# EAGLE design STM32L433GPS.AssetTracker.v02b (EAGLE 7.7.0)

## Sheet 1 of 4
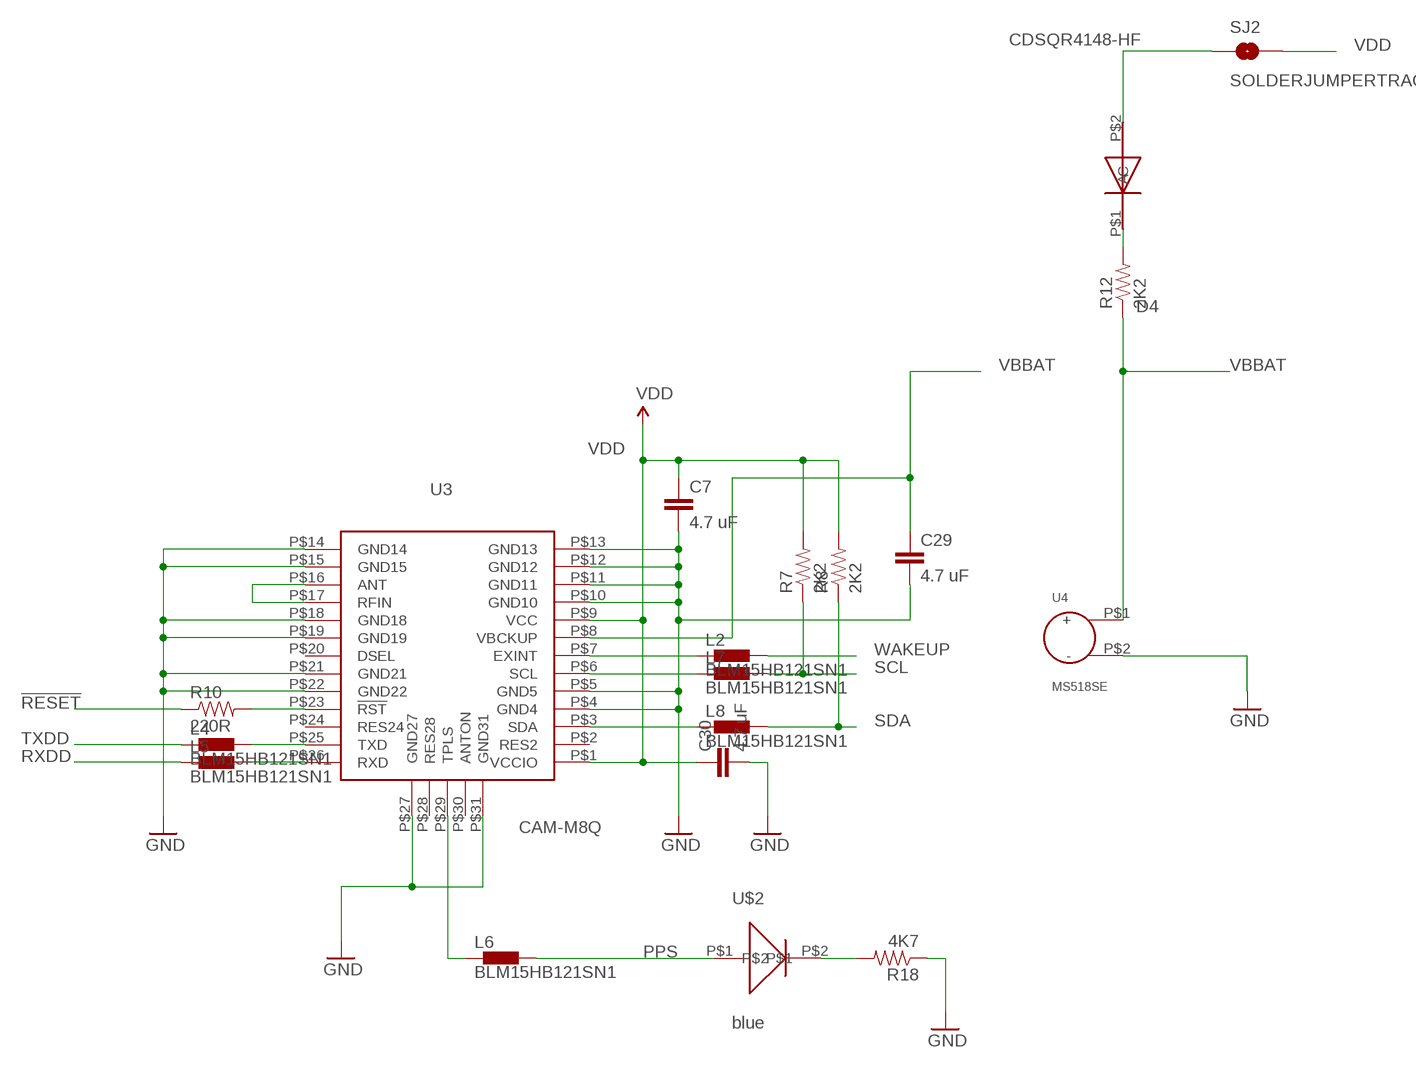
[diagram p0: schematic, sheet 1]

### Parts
C7  4.7 uF  0402CAP.KW  [0402-CAP]
C29  4.7 uF  0402CAP.KW  [0402-CAP]
C30  4.7 uF  0402CAP.KW  [0402-CAP]
D4  CDSQR4148-HF  [CDSQR4148-HF]
L2  BLM15HB121SN1  [0402]
L4  BLM15HB121SN1  [0402]
L5  BLM15HB121SN1  [0402]
L6  BLM15HB121SN1  [0402]
L7  BLM15HB121SN1  [0402]
L8  BLM15HB121SN1  [0402]
R7  2K2  0402RES.KW  [0402-RES]
R8  2K2  0402RES.KW  [0402-RES]
R10  220R  0402RES.KW  [0402-RES]
R12  2K2  0402RES.KW  [0402-RES]
R18  4K7  0402RES.KW  [0402-RES]
SJ2  SOLDERJUMPERTRACE  [SJ_2S-TRACE]
U3  CAM-M8Q  [CAM-M8Q]
U4  MS518SE  [MS518SE]
U$2  blue  0402LED  [0402LED]

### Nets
!RESET: R10.1
GND: C7.2 C29.2 C30.2 R18.1 U3.P$4(GND4) U3.P$5(GND5) U3.P$10(GND10) U3.P$11(GND11) U3.P$12(GND12) U3.P$13(GND13) U3.P$14(GND14) U3.P$15(GND15) U3.P$18(GND18) U3.P$19(GND19) U3.P$21(GND21) U3.P$22(GND22) U3.P$27(GND27) U3.P$31(GND31) U4.P$2(-) ; also sheet 2,3,4
N$4: D4.P$2(A) SJ2.1
N$5: D4.P$1(C) R12.2
N$6: L2.1 U3.P$7(EXINT)
N$8: R18.2 U$2.P$2
N$10: L7.1 U3.P$6(SCL)
N$23: L8.1 U3.P$3(SDA)
N$43: L4.2 U3.P$25(TXD)
N$44: L5.2 U3.P$26(RXD)
N$45: U3.P$16(ANT) U3.P$17(RFIN)
N$46: R10.2 U3.P$23(!RST)
N$47: L6.1 U3.P$29(TPLS)
PPS: L6.2 U$2.P$1 ; also sheet 4
RXDD: L5.1 ; also sheet 4
SCL: L7.2 R7.1 ; also sheet 3,4
SDA: L8.2 R8.1 ; also sheet 3,4
TXDD: L4.1 ; also sheet 4
VBBAT: C29.1 R12.1 U3.P$8(VBCKUP) U4.P$1(+)
VDD: C7.1 C30.1 R7.2 R8.2 SJ2.2 U3.P$1(VCCIO) U3.P$9(VCC) ; also sheet 2,3,4
WAKEUP: L2.2 ; also sheet 4
Unconnected: U3.P$2(RES2) U3.P$20(DSEL) U3.P$24(RES24) U3.P$28(RES28) U3.P$30(ANTON)

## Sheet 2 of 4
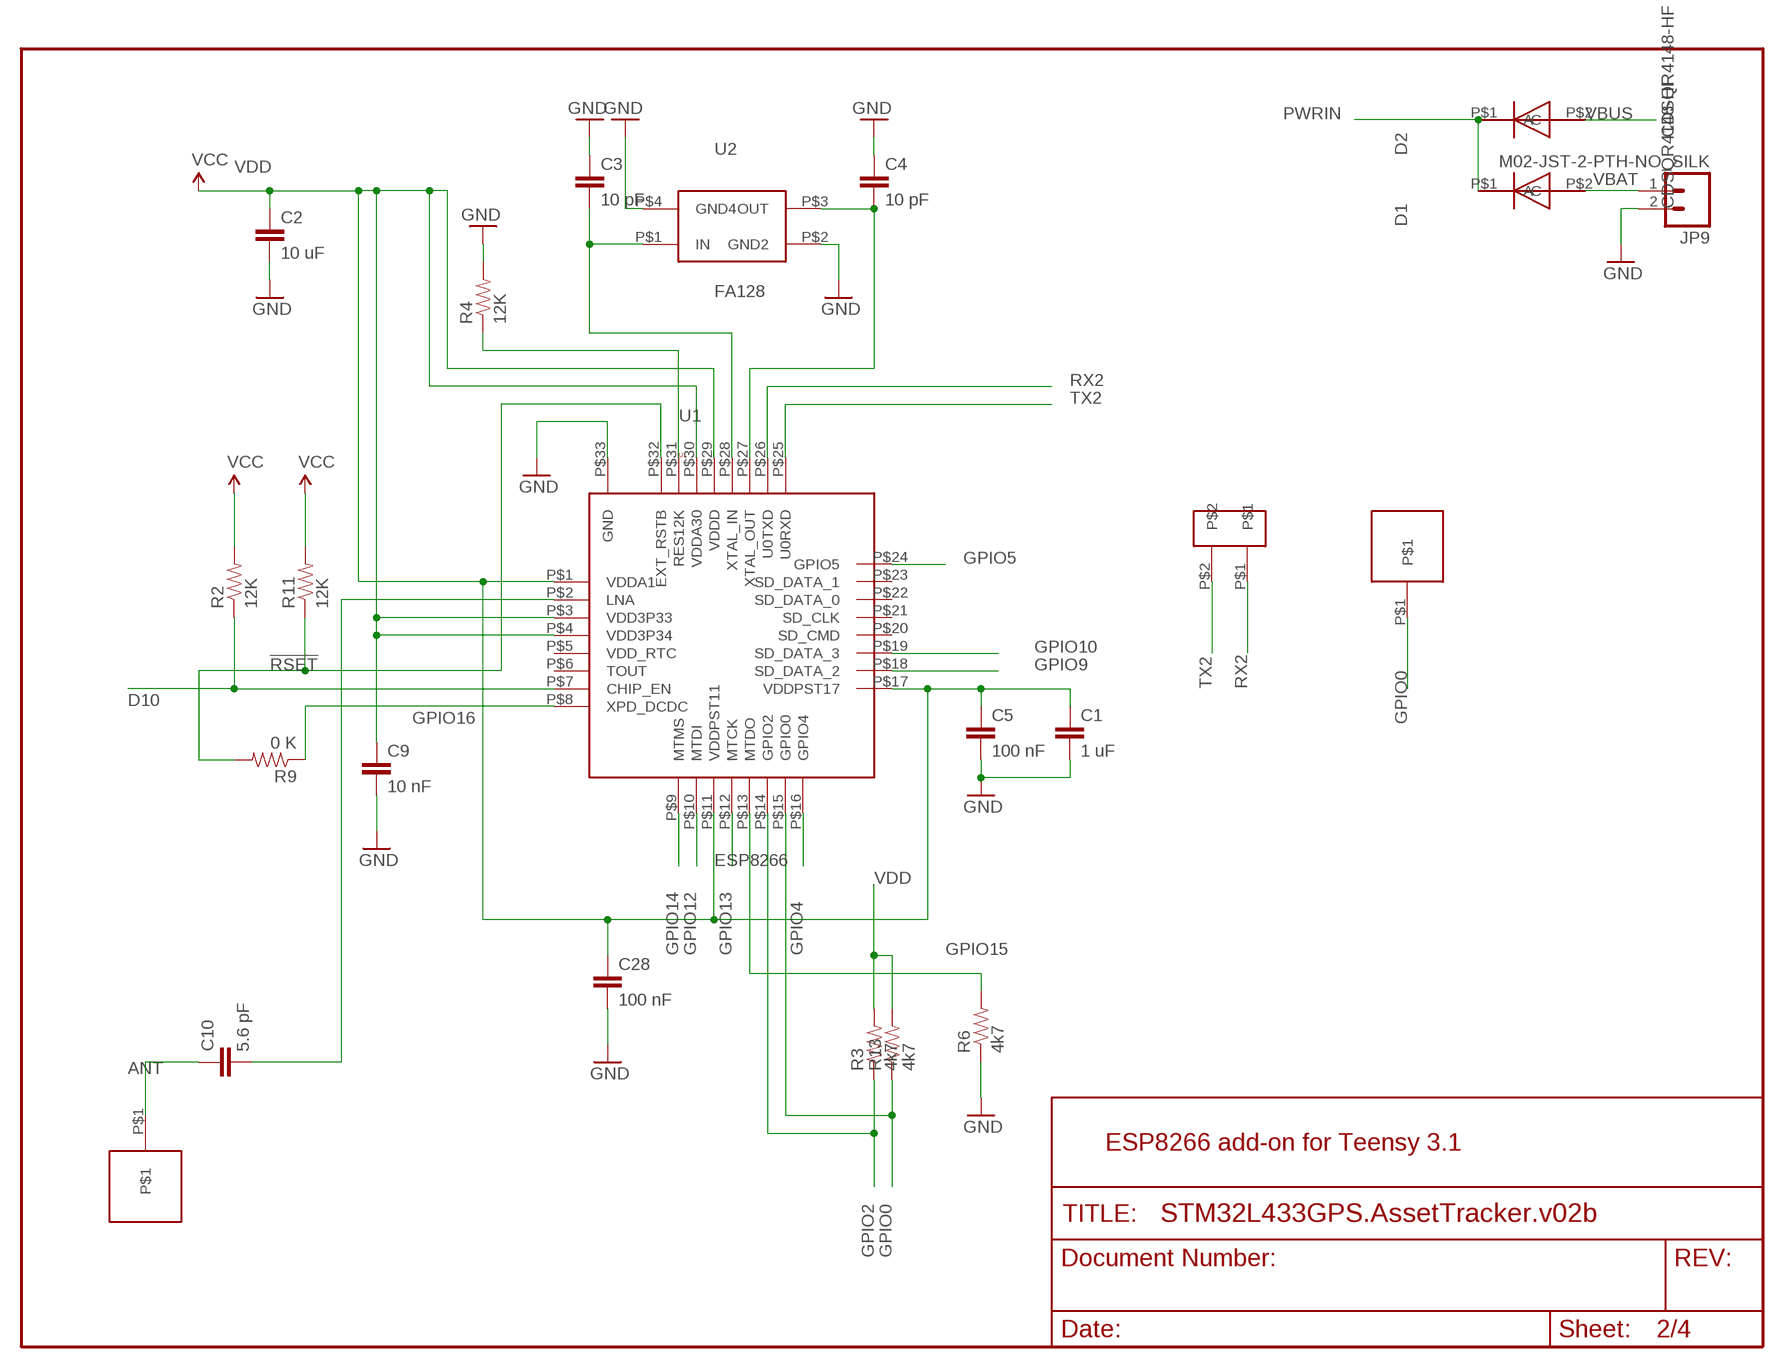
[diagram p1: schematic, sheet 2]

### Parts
C1  1 uF  0402CAP.KW  [0402-CAP]
C2  10 uF  0402CAP.KW  [0402-CAP]
C3  10 pF  0402CAP.KW  [0402-CAP]
C4  10 pF  0402CAP.KW  [0402-CAP]
C5  100 nF  0402CAP.KW  [0402-CAP]
C9  10 nF  0402CAP.KW  [0402-CAP]
C10  5.6 pF  0402CAP.KW  [0402-CAP]
C28  100 nF  0402CAP.KW  [0402-CAP]
D1  CDSQR4148-HF  [CDSQR4148-HF]
D2  CDSQR4148-HF  [CDSQR4148-HF]
JP9  M02-JST-2-PTH-NO_SILK  [JST-2-PTH-NS]
R2  12K  0402RES.KW  [0402-RES]
R3  4k7  0402RES.KW  [0402-RES]
R4  12K  0402RES.KW  [0402-RES]
R6  4k7  0402RES.KW  [0402-RES]
R9  0 K  0402RES.KW  [0402-RES]
R11  12K  0402RES.KW  [0402-RES]
R13  4k7  0402RES.KW  [0402-RES]
U1  ESP8266  [ESP8266]
U2  FA128  [FA128]
U$1  HN02  [HN02]
U$3  HN01  [HN01]
U$15  HN01  [HN01]

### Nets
!RSET: R9.2 R11.1 U1.P$32(EXT_RSTB)
ANT: C10.1 U$15.P$1
D10: R2.1 U1.P$7(CHIP_EN) ; also sheet 4
GND: C1.2 C2.2 C3.1 C4.1 C5.2 C9.2 C28.2 JP9.2 R4.2 R6.1 U1.P$33(GND) U2.P$2(GND2) U2.P$4(GND4) ; also sheet 1,3,4
GPIO0: R13.1 U1.P$15(GPIO0) U$3.P$1
GPIO2: R3.1 U1.P$14(GPIO2)
GPIO4: U1.P$16(GPIO4)
GPIO5: U1.P$24(GPIO5)
GPIO9: U1.P$18(SD_DATA_2)
GPIO10: U1.P$19(SD_DATA_3)
GPIO12: U1.P$10(MTDI)
GPIO13: U1.P$12(MTCK)
GPIO14: U1.P$9(MTMS)
GPIO15: R6.2 U1.P$13(MTDO)
GPIO16: R9.1 U1.P$8(XPD_DCDC)
N$1: C3.2 U1.P$28(XTAL_IN) U2.P$1(IN)
N$2: C4.2 U1.P$27(XTAL_OUT) U2.P$3(OUT)
N$3: C10.2 U1.P$2(LNA)
N$13: R4.1 U1.P$31(RES12K)
PWRIN: D1.P$1(C) D2.P$1(C) ; also sheet 4
RX2: U1.P$26(U0TXD) U$1.P$1 ; also sheet 4
TX2: U1.P$25(U0RXD) U$1.P$2 ; also sheet 4
VBAT: D1.P$2(A) JP9.1 ; also sheet 4
VBUS: D2.P$2(A) ; also sheet 4
VDD: C1.1 C2.1 C5.1 C9.1 C28.1 R2.2 R3.2 R11.2 R13.2 U1.P$1(VDDA1) U1.P$3(VDD3P33) U1.P$4(VDD3P34) U1.P$11(VDDPST11) U1.P$17(VDDPST17) U1.P$29(VDDD) U1.P$30(VDDA30) ; supply symbol labelled VCC ; also sheet 1,3,4
Unconnected: U1.P$5(VDD_RTC) U1.P$6(TOUT) U1.P$20(SD_CMD) U1.P$21(SD_CLK) U1.P$22(SD_DATA_0) U1.P$23(SD_DATA_1)

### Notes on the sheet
- ESP8266 add-on for Teensy 3.1

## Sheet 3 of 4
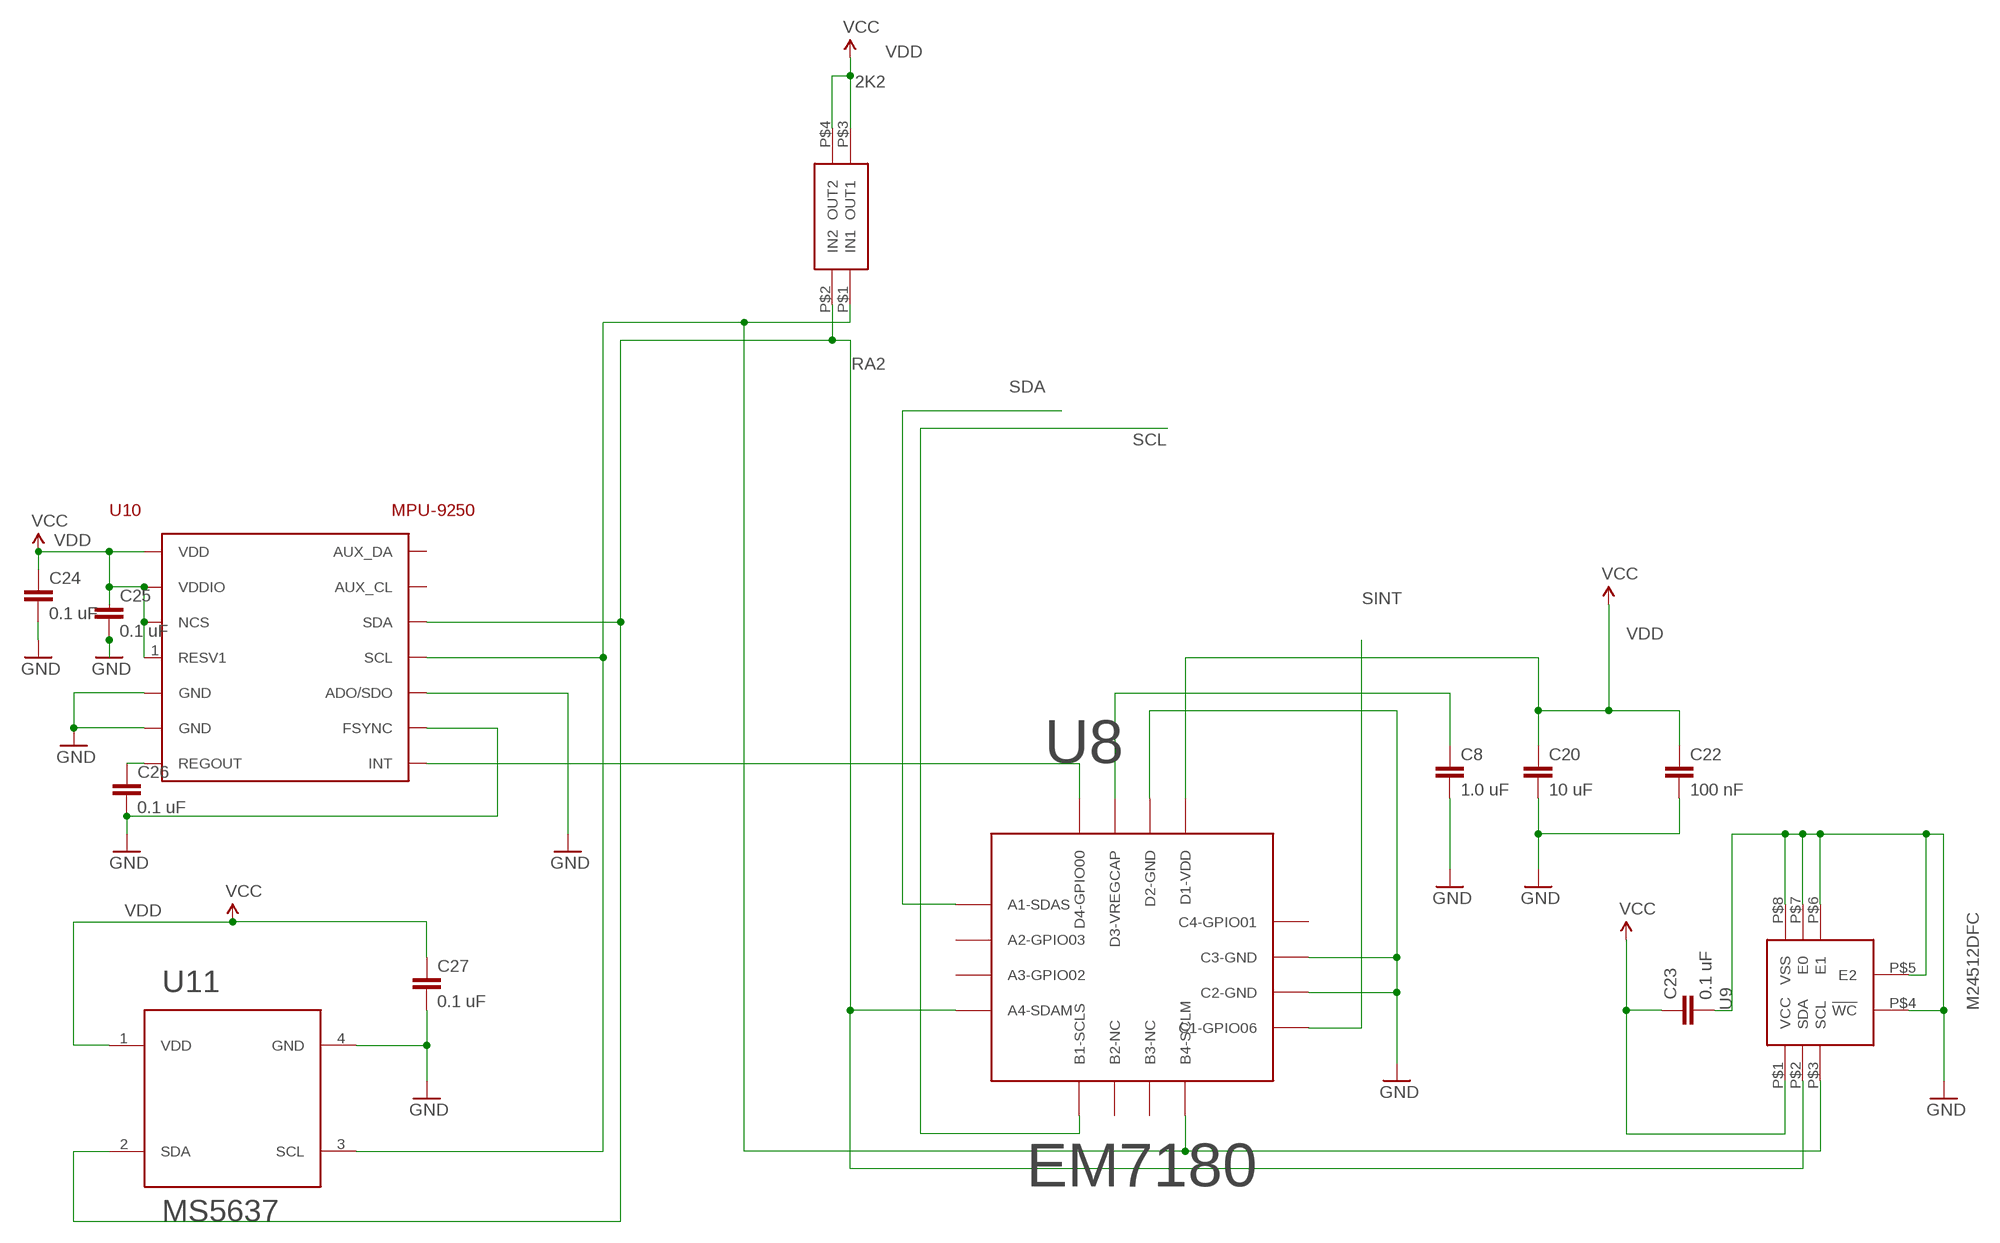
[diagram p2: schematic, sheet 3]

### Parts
C8  1.0 uF  CAP0402-CAP  [0402-CAP]
C20  10 uF  CAP0402-CAP  [0402-CAP]
C22  100 nF  CAP0402-CAP  [0402-CAP]
C23  0.1 uF  CAP0402-CAP  [0402-CAP]
C24  0.1 uF  CAP0402-CAP  [0402-CAP]
C25  0.1 uF  CAP0402-CAP  [0402-CAP]
C26  0.1 uF  CAP0402-CAP  [0402-CAP]
C27  0.1 uF  CAP0402-CAP  [0402-CAP]
RA2  2K2  EXB24V  [EXB24V]
U8  EM7180  [WL-CSP16]
U9  M24512DFC  [M24512DFC]
U10  MPU-9250  [MPU-9250]
U11  MS5637  [MS5637QFN-4]

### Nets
GND: C8.2 C20.2 C22.2 C23.2 C24.2 C25.2 C26.2 C27.2 U8.P$10(C2-GND) U8.P$11(C3-GND) U8.P$14(D2-GND) U9.P$4(!WC) U9.P$5(E2) U9.P$6(E1) U9.P$7(E0) U9.P$8(VSS) U10.9(ADO/SDO) U10.11(FSYNC) U10.18(GND) U10.20(GND) U11.4(GND) ; also sheet 1,2,4
N$19: U8.P$16(D4-GPIO00) U10.12(INT)
N$26: C8.1 U8.P$15(D3-VREGCAP)
N$40: C26.1 U10.10(REGOUT)
SCL: U8.P$5(B1-SCLS) ; also sheet 1,4
SCL2: RA2.P$1(IN1) U8.P$8(B4-SCLM) U9.P$3(SCL) U10.23(SCL) U11.3(SCL)
SDA: U8.P$1(A1-SDAS) ; also sheet 1,4
SDA2: RA2.P$2(IN2) U8.P$4(A4-SDAM) U9.P$2(SDA) U10.24(SDA) U11.2(SDA)
SINT: U8.P$9(C1-GPIO06) ; also sheet 4
VDD: C20.1 C22.1 C23.1 C24.1 C25.1 C27.1 RA2.P$3(OUT1) RA2.P$4(OUT2) U8.P$13(D1-VDD) U9.P$1(VCC) U10.1(RESV1) U10.8(VDDIO) U10.13(VDD) U10.22(NCS) U11.1(VDD) ; supply symbol labelled VCC ; also sheet 1,2,4
Unconnected: U8.P$2(A2-GPIO03) U8.P$3(A3-GPIO02) U8.P$6(B2-NC) U8.P$7(B3-NC) U8.P$12(C4-GPIO01) U10.7(AUX_CL) U10.21(AUX_DA)

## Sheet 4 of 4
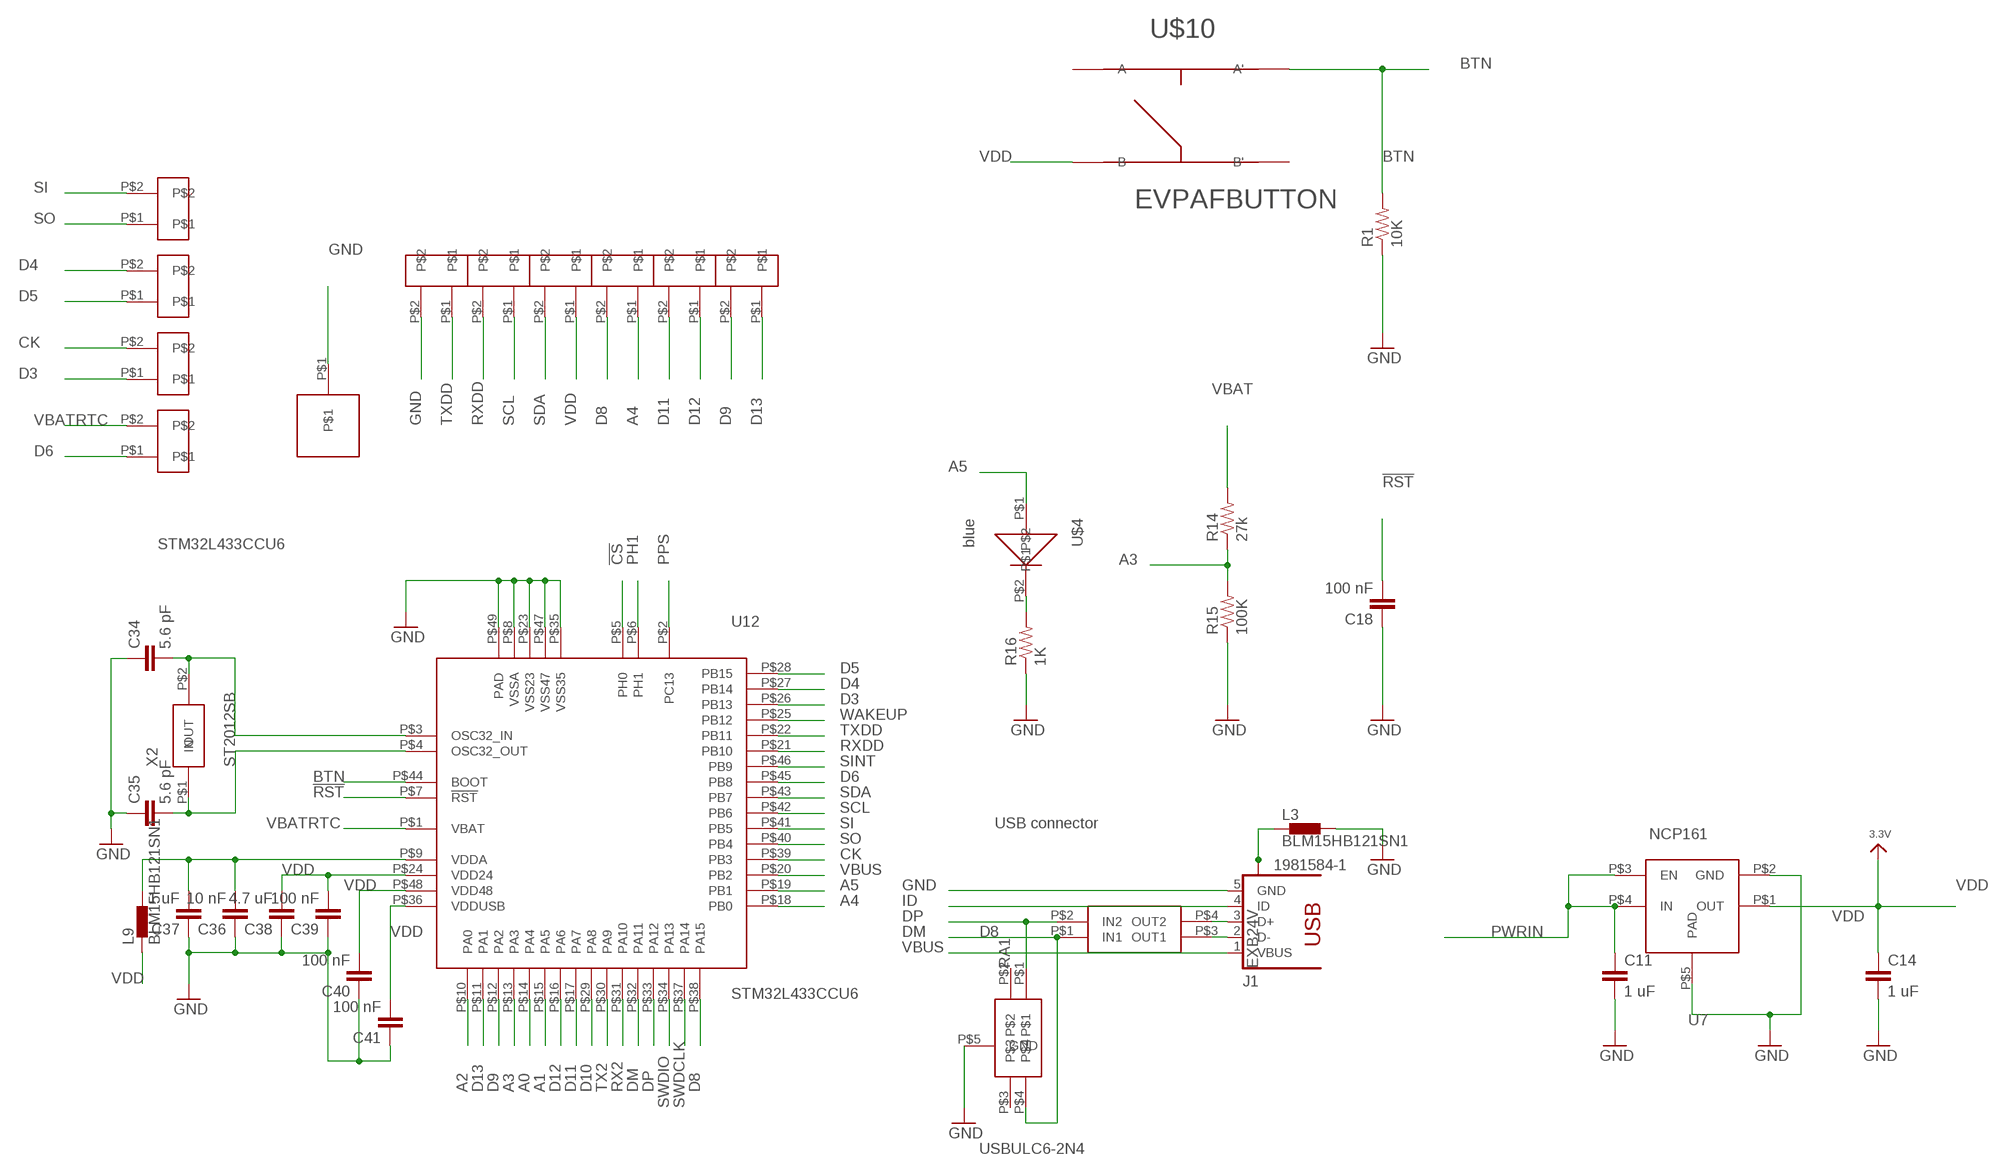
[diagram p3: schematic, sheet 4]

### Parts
C11  1 uF  CAP0402-CAP  [0402-CAP]
C14  1 uF  CAP0402-CAP  [0402-CAP]
C18  100 nF  0402CAP.KW  [0402-CAP]
C34  5.6 pF  0402CAP.KW  [0402-CAP]
C35  5.6 pF  0402CAP.KW  [0402-CAP]
C36  10 nF  0402CAP.KW  [0402-CAP]
C37  1 uF  0402CAP.KW  [0402-CAP]
C38  4.7 uF  0402CAP.KW  [0402-CAP]
C39  100 nF  0402CAP.KW  [0402-CAP]
C40  100 nF  0402CAP.KW  [0402-CAP]
C41  100 nF  0402CAP.KW  [0402-CAP]
D8  USBULC6-2N4  [USBULC6-2N4]
J1  1981584-1  [1981584-1]
L3  BLM15HB121SN1  [0402]
L9  BLM15HB121SN1  [0402]
R1  10K  0402RES.KW  [0402-RES]
R14  27k  0402RES.KW  [0402-RES]
R15  100K  0402RES.KW  [0402-RES]
R16  1K  0402RES.KW  [0402-RES]
RA1  EXB24V  [EXB24V]
U7  NCP161  [NCP161]
U12  STM32L433CCU6  [STM32L433CCU6]
U$4  blue  0402LED  [0402LED]
U$10  EVPAFBUTTON  [EVPAF-BUTTON-SPDT]
U$11  HN02  [HN02]
U$12  HN02  [HN02]
U$13  HN02  [HN02]
U$14  HN02  [HN02]
U$16  HN02  [HN02]
U$17  HN02  [HN02]
U$19  HN01  [HN01]
U$30  HN02  [HN02]
U$31  HN02  [HN02]
U$32  HN02  [HN02]
U$36  HN02  [HN02]
X2  ST2012SB  [ST2012SB]

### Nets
!CS: U12.P$5(PH0)
!RST: C18.2 U12.P$7(!RST)
A0: U12.P$14(PA4)
A1: U12.P$15(PA5)
A2: U12.P$10(PA0)
A3: R14.1 R15.2 U12.P$13(PA3)
A4: U12.P$18(PB0) U$14.P$1
A5: U12.P$19(PB1) U$4.P$1
BTN: R1.2 U12.P$44(BOOT) U$10.P$2(A')
CK: U12.P$39(PB3) U$31.P$2
D3: U12.P$26(PB13) U$31.P$1
D4: U12.P$27(PB14) U$32.P$2
D5: U12.P$28(PB15) U$32.P$1
D6: U12.P$45(PB8) U$36.P$1
D8: U12.P$38(PA15) U$14.P$2
D9: U12.P$12(PA2) U$16.P$2
D10: U12.P$29(PA8) ; also sheet 2
D11: U12.P$17(PA7) U$17.P$2
D12: U12.P$16(PA6) U$17.P$1
D13: U12.P$11(PA1) U$16.P$1
DM: D8.P$4 RA1.P$1(IN1) U12.P$32(PA11)
DP: D8.P$1 RA1.P$2(IN2) U12.P$33(PA12)
GND: C11.2 C14.2 C18.1 C34.1 C35.1 C36.1 C37.1 C38.1 C39.1 C40.1 C41.1 D8.P$5(GND) J1.5(GND) L3.2 R1.1 R15.1 R16.1 U7.P$2(GND) U7.P$5(PAD) U12.P$8(VSSA) U12.P$23(VSS23) U12.P$35(VSS35) U12.P$47(VSS47) U12.P$49(PAD) U$11.P$2 U$19.P$1 ; also sheet 1,2,3
ID: J1.4(ID)
N$9: C34.2 U12.P$3(OSC32_IN) X2.P$2(OUT)
N$11: R16.2 U$4.P$2
N$12: C35.2 U12.P$4(OSC32_OUT) X2.P$1(IN)
N$17: C36.2 C37.2 L9.2 U12.P$9(VDDA)
N$31: J1.3(D+) RA1.P$4(OUT2)
N$33: J1.2(D-) RA1.P$3(OUT1)
PH1: U12.P$6(PH1)
PPS: U12.P$2(PC13) ; also sheet 1
PWRIN: C11.1 U7.P$3(EN) U7.P$4(IN) ; also sheet 2
RX2: U12.P$31(PA10) ; also sheet 2
RXDD: U12.P$21(PB10) U$12.P$2 ; also sheet 1
SCL: U12.P$42(PB6) U$12.P$1 ; also sheet 1,3
SDA: U12.P$43(PB7) U$13.P$2 ; also sheet 1,3
SI: U12.P$41(PB5) U$30.P$2
SINT: U12.P$46(PB9) ; also sheet 3
SO: U12.P$40(PB4) U$30.P$1
SWDCLK: U12.P$37(PA14)
SWDIO: U12.P$34(PA13)
TX2: U12.P$30(PA9) ; also sheet 2
TXDD: U12.P$22(PB11) U$11.P$1 ; also sheet 1
USB_SHIELD1: J1.S1 J1.S2 J1.S3 J1.S4 L3.1
VBAT: R14.2 ; also sheet 2
VBATRTC: U12.P$1(VBAT) U$36.P$2
VBUS: J1.1(VBUS) U12.P$20(PB2) ; also sheet 2
VDD: C14.1 C38.2 C39.2 C40.2 C41.2 L9.1 U7.P$1(OUT) U12.P$24(VDD24) U12.P$36(VDDUSB) U12.P$48(VDD48) U$10.P$3(B) U$13.P$1 ; supply symbol labelled 3.3V ; also sheet 1,2,3
WAKEUP: U12.P$25(PB12) ; also sheet 1
Unconnected: D8.P$2 D8.P$3 U$10.P$1(A) U$10.P$4(B')

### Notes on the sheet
- STM32L433CCU6
- USB connector

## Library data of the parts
C1-C5 C7 C9 C10 C18 C28-C30 C34-C41 = SparkFun-Capacitors:0402CAP.KW
C8 C11 C14 C20 C22-C27 = SparkFun-Capacitors:CAP: Capacitor
D1 D2 D4 = Kris:CDSQR4148-HF: ComChip's CDSQR4148-HF high speed 150 mA Io diode
D8 = Kris:USBULC6-2N4: ST TVS diode ESD Protection USBULC6-2N4
J1 = con-usb:1981584-1: Receptacle, micro-USB, type A/B Tyco Electronics; MF: Hirose; MPN: ZX62-AB-5PA(11)
JP9 = SparkFun-Connectors:M02: Standard 2-pin 0.1" header. Use with
L2-L9 = inductors:BLM15H: EMIFIL (R) Chip Ferrite Bead for GHz Noise
R1-R4 R6-R16 R18 = SparkFun-Resistors:0402RES.KW
RA1 RA2 = Kris:EXB24V: Panasonic EXB24 22 Ohm series resistor pair
SJ2 = SparkFun-Passives:SOLDERJUMPER: Solder Jumper
U1 = Kris:ESP8266: QFN-32 package for espressif's ESP8266 WiFi microprocessor
U2 = Kris:FA128: FA-128 Espon crystal
U3 = ubloxLib:CAM-M8Q: CAM-M8Q GPS/GNSS Module https://www.u-blox.com/sites/default/files/CAM-M8_HardwareIntegrationManual_%28UBX-14000014%29.pdf
U4 = Kris:MS518SE: S518SE 3 V rechargable Li battery
U7 = Kris:NCP161: NCP161 3V3 LDO voltage regulator
U8 = SparkFun-DigitalIC:EM7180: WL-CSP19 package for the EM7180 SENtral sensor fusion hub
U9 = Kris:M24512DFC: ST's M24512DFC6 512 Mbit EEPROM
U10 = SparkFun-Sensors:MPU-9250: The MPU-9250 is a 9-axis motion sensor that contains an accelerometer/gyro sensor (MPU-6500) combined with a magnetometer (AK8963).
U11 = SparkFun-DiscreteSemi:MS5637: MS5637 I2C pressure sensor in QFN-4 package by Measurement Specialties
U12 = STM32L433CCU6:STM32L433CCU6: UFQFPN48 48-lead, 7 mm x 7 mm, 0.5-mm pitch, ultra thin fine pitch quad flat package for STM32L433 http://www.st.com/content/ccc/resource/technical/document/datasheet/f7/a0/fc/27/24/4e/4f/3f/DM00257192.pdf/files/DM00257192.pdf/jcr:content/translations/en.DM00257192.pdf
U$1 U$11-U$14 U$16 U$17 U$30-U$32 U$36 = Kris:HN02: 0.1 inch header
U$2 U$4 = Kris:0402LED: 0402led
U$3 U$15 U$19 = PWSONN6:HN01
U$10 = SparkFun-Electromechanical:EVPAFBUTTON: EVPAF Momentary switch by panasonic
X2 = Kris:ST2012SB: Kyocera 2.0 x 1.2 mm 32.768 20kHz ppm 4 pf crystal

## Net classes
1 USB: width 0.254 mm, drill 0.33 mm, clearance 0.159 mm
2 Top GND Pour: clearance 0.762 mm to class 1

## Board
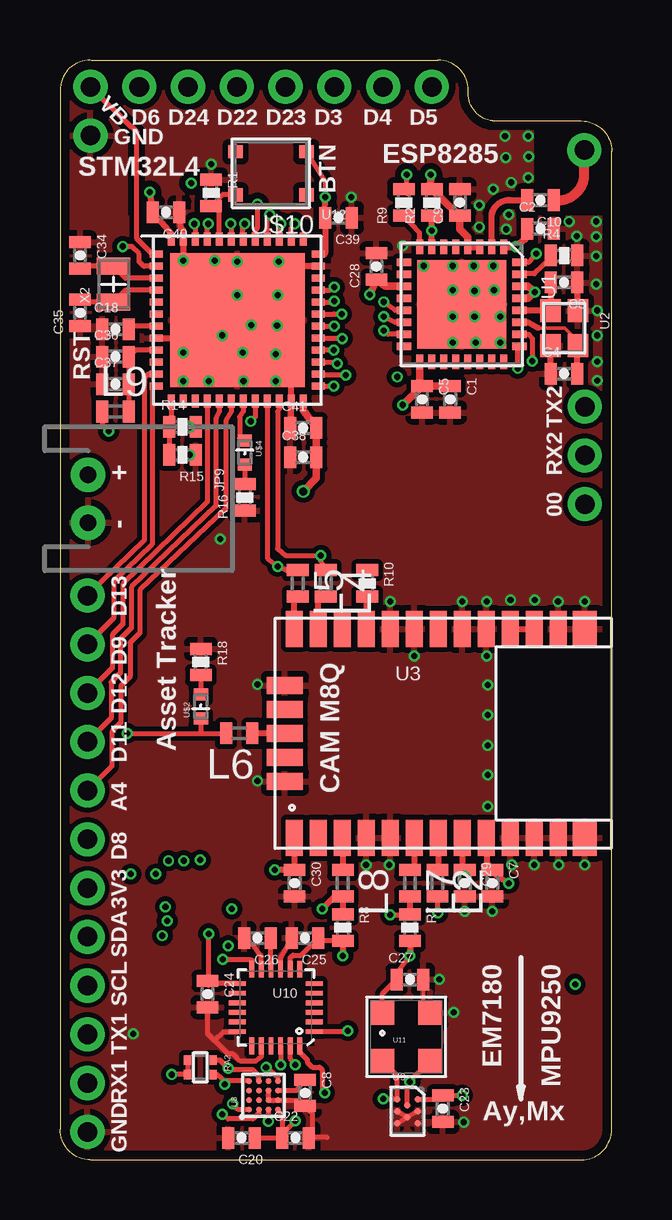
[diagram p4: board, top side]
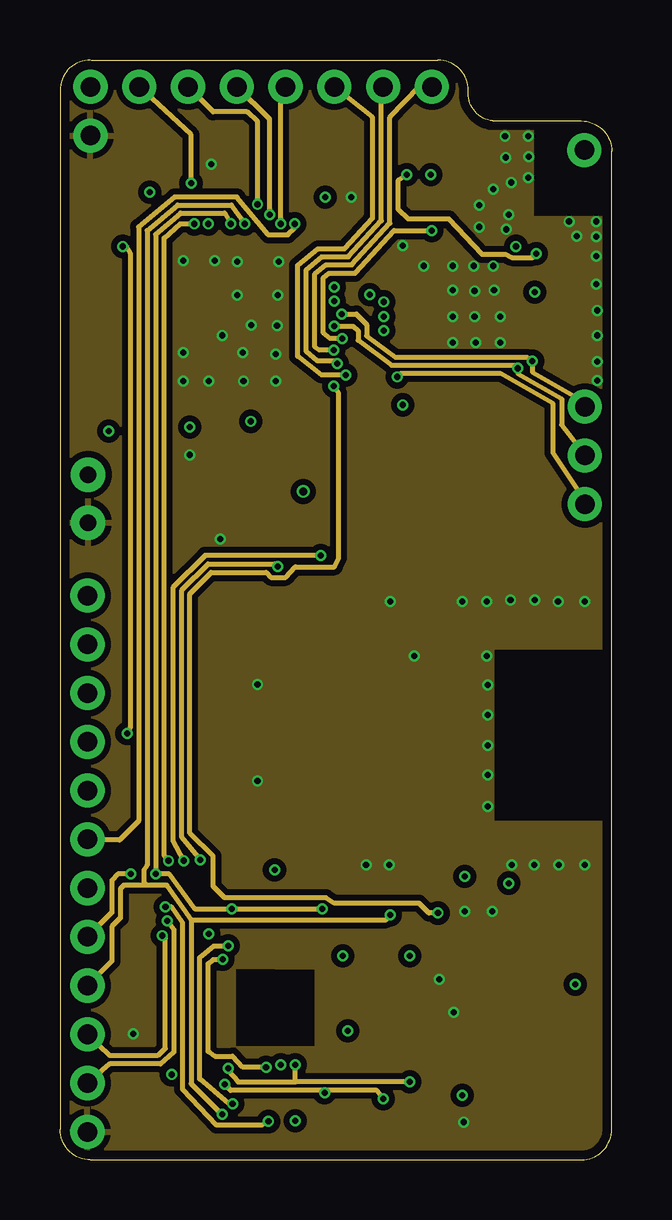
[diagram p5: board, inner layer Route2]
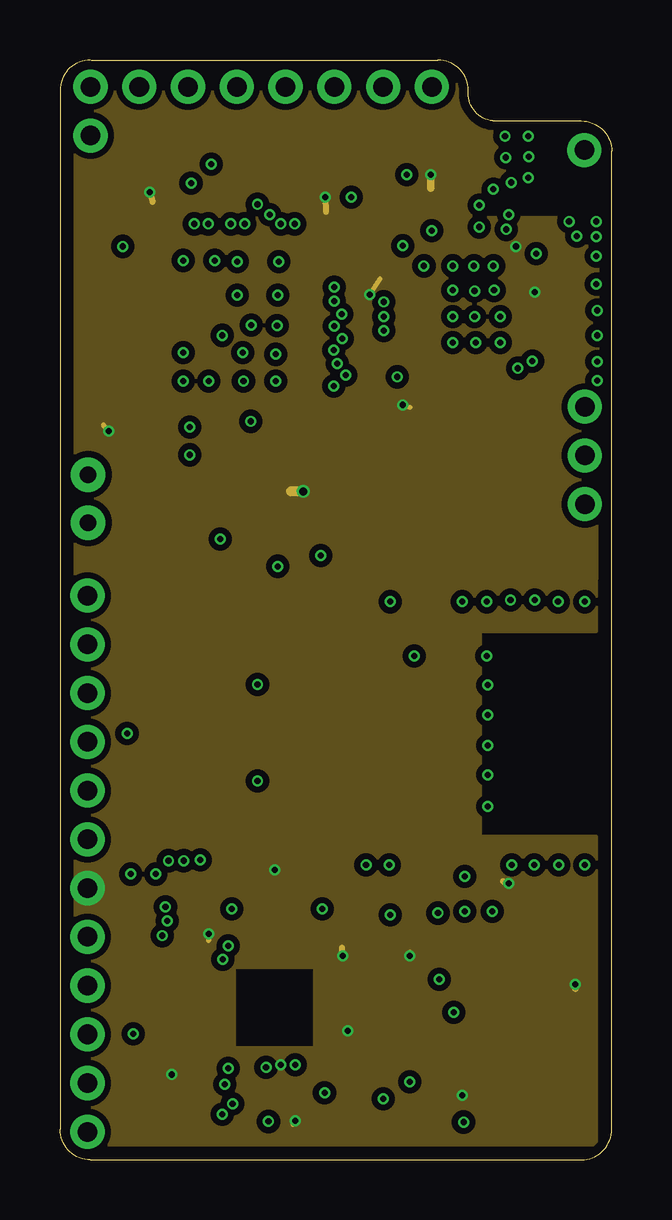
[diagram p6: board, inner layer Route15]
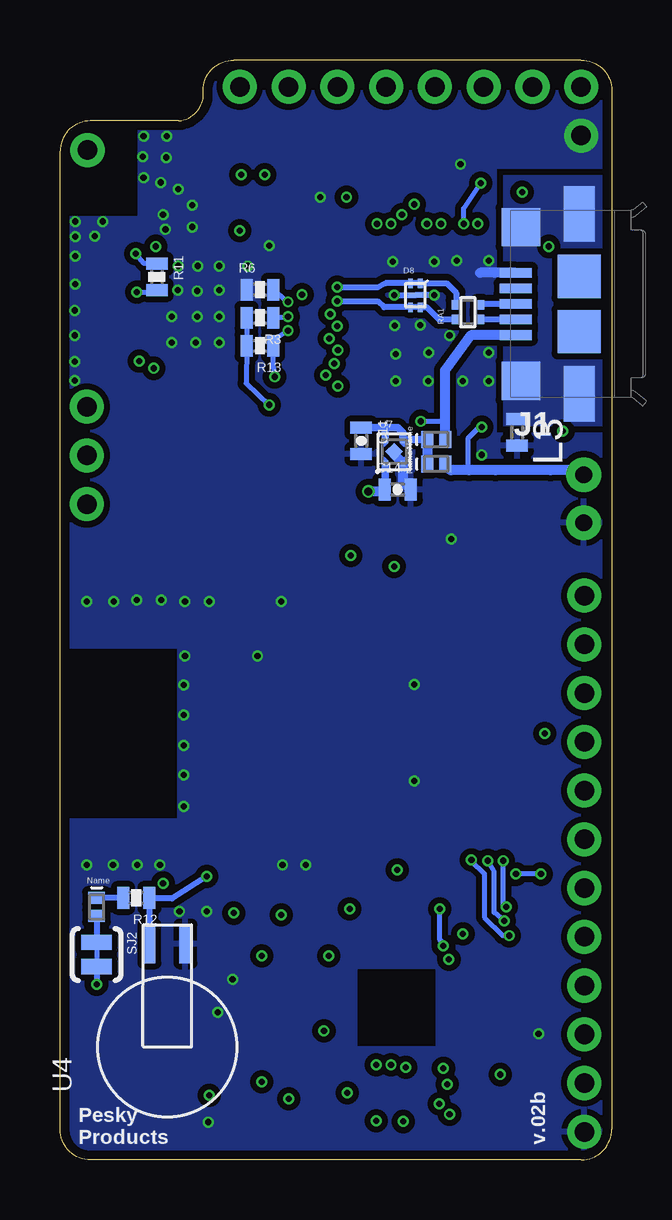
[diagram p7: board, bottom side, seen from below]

Size 22.99 x 45.85 mm. Coordinates in mm from the lower left corner, seen from the top.
Outline: 1.27,45.85 arc90 0,44.58 0,1.27 arc90 1.27,0 21.72,0 arc90 22.99,1.27 22.99,42.04 arc90 21.72,43.31 18.03,43.31 arc-90 17.02,44.58 arc90 15.75,45.85 1.29,45.85
Copper layers (1*2*15*16): Top 0.035559375mm / dielectric 0.17018125mm / Route2 0.01778125mm / dielectric 47mil / Route15 0.01778125mm / dielectric 0.17018125mm / Bottom 0.035559375mm
Design rules "OSHPark-4layer *": minimum track width 5mil, minimum drill 10mil, track to track 5mil, track to pad 5mil, pad to pad 5mil, via to via 5mil, smd to smd 5mil, copper to edge 15mil, drill to drill 6mil, minimum pad ring 4mil, minimum via ring 4mil, stop-mask expansion 4mil, vias tented up to drill 20mil, thermal gap 10mil

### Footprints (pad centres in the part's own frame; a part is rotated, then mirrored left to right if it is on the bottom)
0402-CAP = smd 0.5 x 0.9: 1 -0.55,0; 2 0.55,0
CDSQR4148-HF = smd 0.7 x 0.5: P$1 0,0.375; P$2 0,-0.375
USBULC6-2N4 = smd 0.2 x 0.4: P$1 0.2,0.5; P$2 -0.2,0.5; P$3 -0.2,-0.5; P$4 0.2,-0.5 | smd 0.6 x 0.2: P$5 0,0
1981584-1 = smd 0.4 x 1.35: 1 -1.3,4.1; 2 -0.65,4.1; 3 0,4.1; 4 0.65,4.1; 5 1.3,4.1 | smd 1.8 x 1.8: M1 -1.15,1.45; M2 1.15,1.45 | smd 2.3 x 1.3: S1 -3.75,1.45; S2 3.75,1.45 | smd 1.6 x 1.6: S3 -3.2,3.885; S4 3.2,3.885
JST-2-PTH-NS = drill 0.7 pad 1.448: 1 -1,0; 2 1,0
0402 = smd 0.5 x 0.9: 1 -0.55,0; 2 0.55,0
0402-RES = smd 0.5 x 0.9: 1 -0.55,0; 2 0.55,0
EXB24V = smd 0.4 x 0.36: P$1 -0.3,0.5; P$2 0.3,0.5; P$3 -0.3,-0.5; P$4 0.3,-0.5
SJ_2S-TRACE = smd 0.635 x 1.27: 1 -0.508,0; 2 0.508,0
ESP8266 = smd 0.6 x 0.3: P$1 -2.4,1.75; P$2 -2.4,1.25; P$3 -2.4,0.75; P$4 -2.4,0.25; P$5 -2.4,-0.25; P$6 -2.4,-0.75; P$7 -2.4,-1.25; P$8 -2.4,-1.75; P$17 2.4,-1.75; P$18 2.4,-1.25; P$19 2.4,-0.75; P$20 2.4,-0.25; P$21 2.4,0.25; P$22 2.4,0.75; P$23 2.4,1.25; P$24 2.4,1.75 | smd 0.3 x 0.6: P$9 -1.75,-2.4; P$10 -1.25,-2.4; P$11 -0.75,-2.4; P$12 -0.25,-2.4; P$13 0.25,-2.4; P$14 0.75,-2.4; P$15 1.25,-2.4; P$16 1.75,-2.4; P$25 1.75,2.4; P$26 1.25,2.4; P$27 0.75,2.4; P$28 0.25,2.4; P$29 -0.25,2.4; P$30 -0.75,2.4; P$31 -1.25,2.4; P$32 -1.75,2.4 | smd 3.7 x 3.7: P$33 0,0
FA128 = smd 0.95 x 0.85: P$1 -0.725,-0.575; P$2 0.725,-0.575; P$3 0.725,0.575; P$4 -0.725,0.575
CAM-M8Q = smd 0.7 x 1.5: P$1 0.8,0.45; P$2 1.8,0.45; P$3 2.8,0.45; P$4 3.8,0.45; P$5 4.8,0.45; P$6 5.8,0.45; P$7 6.8,0.45; P$8 7.8,0.45; P$9 8.8,0.45; P$10 9.8,0.45; P$11 10.8,0.45; P$12 11.8,0.45; P$15 11.8,9.15; P$16 10.8,9.15; P$17 9.8,9.15; P$18 8.8,9.15; P$19 7.8,9.15; P$20 6.8,9.15; P$21 5.8,9.15; P$22 4.8,9.15; P$23 3.8,9.15; P$24 2.8,9.15; P$25 1.8,9.15; P$26 0.8,9.15 | smd 1 x 1.5: P$13 12.9,0.45; P$14 12.9,9.15 | smd 1.5 x 0.7: P$27 0.4,6.8; P$28 0.4,5.8; P$29 0.4,4.8; P$30 0.4,3.8; P$31 0.4,2.8
MS518SE = smd 1.6 x 0.5: P$1 4.3,0.75; P$2 4.3,-0.75
NCP161 = smd 0.24 x 0.24: P$1 -0.37,-0.48; P$2 0.37,-0.48; P$3 0.37,0.48; P$4 -0.37,0.48 | smd 0.52 x 0.52 rotated 45: P$5 0,0
WL-CSP16 = smd 0.24 x 0.24: P$1 -0.6,0.6; P$2 -0.2,0.6; P$3 0.2,0.6; P$4 0.6,0.6; P$5 -0.6,0.2; P$6 -0.2,0.2; P$7 0.2,0.2; P$8 0.6,0.2; P$9 -0.6,-0.2; P$10 -0.2,-0.2; P$11 0.2,-0.2; P$12 0.6,-0.2; P$13 -0.6,-0.6; P$14 -0.2,-0.6; P$15 0.2,-0.6; P$16 0.6,-0.6
M24512DFC = smd 0.27 x 0.27: P$1 0.433,0.5; P$2 -0.433,0.5; P$3 0,0.25; P$4 0.433,0; P$5 -0.433,0; P$6 0,-0.25; P$7 0.433,-0.5; P$8 -0.433,-0.5
MPU-9250 = smd 0.7 x 0.2: 1 -1.6,1; 2 -1.6,0.6; 3 -1.6,0.2; 4 -1.6,-0.2; 5 -1.6,-0.6; 6 -1.6,-1; 13 1.6,-1; 14 1.6,-0.6; 15 1.6,-0.2; 16 1.6,0.2; 17 1.6,0.6; 18 1.6,1 | smd 0.2 x 0.7: 7 -1,-1.6; 8 -0.6,-1.6; 9 -0.2,-1.6; 10 0.2,-1.6; 11 0.6,-1.6; 12 1,-1.6; 19 1,1.6; 20 0.6,1.6; 21 0.2,1.6; 22 -0.2,1.6; 23 -0.6,1.6; 24 -1,1.6
MS5637QFN-4 = smd 1 x 1: 1 -1,1; 2 -1,-1; 3 1,-1; 4 1,1
STM32L433CCU6 = smd 0.55 x 0.3: P$1 -3.375,2.75; P$2 -3.375,2.25; P$3 -3.375,1.75; P$4 -3.375,1.25; P$5 -3.375,0.75; P$6 -3.375,0.25; P$7 -3.375,-0.25; P$8 -3.375,-0.75; P$9 -3.375,-1.25; P$10 -3.375,-1.75; P$11 -3.375,-2.25; P$12 -3.375,-2.75; P$25 3.375,-2.75; P$26 3.375,-2.25; P$27 3.375,-1.75; P$28 3.375,-1.25; P$29 3.375,-0.75; P$30 3.375,-0.25; P$31 3.375,0.25; P$32 3.375,0.75; P$33 3.375,1.25; P$34 3.375,1.75; P$35 3.375,2.25; P$36 3.375,2.75 | smd 0.3 x 0.55: P$13 -2.75,-3.375; P$14 -2.25,-3.375; P$15 -1.75,-3.375; P$16 -1.25,-3.375; P$17 -0.75,-3.375; P$18 -0.25,-3.375; P$19 0.25,-3.375; P$20 0.75,-3.375; P$21 1.25,-3.375; P$22 1.75,-3.375; P$23 2.25,-3.375; P$24 2.75,-3.375; P$37 2.75,3.375; P$38 2.25,3.375; P$39 1.75,3.375; P$40 1.25,3.375; P$41 0.75,3.375; P$42 0.25,3.375; P$43 -0.25,3.375; P$44 -0.75,3.375; P$45 -1.25,3.375; P$46 -1.75,3.375; P$47 -2.25,3.375; P$48 -2.75,3.375 | smd 5.6 x 5.6: P$49 0,0
HN02 = drill 0.813 pad 1.422: P$1 0,0; P$2 -2.032,0
0402LED = smd 0.5 x 0.6: P$1 -0.5,0; P$2 0.5,0
HN01 = drill 0.813 pad 1.422: P$1 0,0
EVPAF-BUTTON-SPDT = smd 0.6 x 0.55: P$1 -1.475,0.9; P$2 1.475,0.9; P$3 -1.475,-0.9; P$4 1.475,-0.9
ST2012SB = smd 0.7 x 1.4: P$1 -0.75,0; P$2 0.75,0

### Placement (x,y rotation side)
C1  16.26,31.7 270 top
C2  20.02,38.81 0 top
C3  21.01,36.58 180 top
C4  21.01,32.77 0 top
C5  15.09,31.7 270 top
C7  18.01,11.53 270 top
C8  10.21,2.79 270 top
C9  16.66,39.9 90 top
C10  20.02,40.01 180 top
C11  10.44,29.97 270 bottom
C14  8.92,27.94 0 bottom
C18  2.31,34.62 0 top
C20  7.57,0.91 180 top
C22  9.8,0.91 0 top
C23  15.95,2.13 270 top
C24  6.15,6.91 270 top
C25  10.21,9.25 180 top
C26  8.23,9.25 180 top
C27  14.58,7.52 0 top
C28  13.18,37.24 90 top
C29  16.87,11.53 270 top
C30  9.78,11.53 270 top
C34  0.84,37.69 270 top
C35  0.84,35.31 90 top
C36  2.31,33.48 0 top
C37  2.31,32.33 0 top
C38  10.13,29.29 0 top
C39  11.61,39.27 180 top
C40  4.42,39.5 180 top
C41  10.13,30.51 0 top
D1  7.32,29.01 90 bottom
D2  7.32,30.02 90 bottom
D4  21.46,10.54 0 bottom
D8  8.18,36.04 0 bottom
J1  -0.1,35.68 90 bottom
JP9  1.17,27.56 270 top
L2  15.72,11.53 270 top
L3  3.94,30.33 270 bottom
L4  11.07,24.03 270 top
L5  9.91,24.03 270 top
L6  7.47,17.78 180 top
L7  14.58,11.53 270 top
L8  11.79,11.53 270 top
L9  2.31,31.19 0 top
R1  6.3,40.31 270 top
R2  15.49,39.9 90 top
R3  14.66,35.1 180 bottom
R4  21.01,37.69 0 top
R6  14.66,36.27 0 bottom
R7  14.58,9.68 270 top
R8  11.79,9.68 270 top
R9  14.33,39.9 90 top
R10  12.8,24.03 270 top
R11  18.95,36.8 270 bottom
R12  19.81,10.92 180 bottom
R13  14.66,33.93 180 bottom
R14  5.11,30.56 0 top
R15  5.11,29.39 180 top
R16  7.7,27.61 90 top
R18  5.87,20.75 270 top
RA1  5.99,35.33 90 bottom
RA2  5.84,3.86 270 top
SJ2  21.46,8.56 270 bottom
U1  16.74,35.66 270 top
U2  21.01,34.67 270 top
U3  8.97,12.98 0 top
U4  18.52,4.7 90 bottom
U7  9.07,29.51 0 bottom
U8  8.48,2.69 90 top
U9  14.48,2.03 0 top
U10  8.99,6.35 180 top
U11  14.43,5.13 0 top
U12  7.39,35 0 top
U$1  21.87,31.39 90 top
U$2  5.87,18.9 90 top
U$3  21.87,27.33 0 top
U$4  7.7,29.49 270 top
U$10  8.79,41.12 180 top
U$11  1.14,3.2 90 top
U$12  1.14,7.26 90 top
U$13  1.14,11.33 90 top
U$14  1.14,15.39 90 top
U$15  21.84,42.09 90 top
U$16  1.14,23.52 90 top
U$17  1.14,19.46 90 top
U$19  1.27,42.7 0 top
U$30  7.37,44.73 0 top
U$31  11.43,44.73 0 top
U$32  15.49,44.73 0 top
U$36  3.3,44.73 0 top
X2  2.24,36.5 90 top

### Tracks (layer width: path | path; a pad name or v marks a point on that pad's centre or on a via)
!RSET  (via drill 0.25)
  Top 0.203: v19.84,37.77 19.52,37.41 U1.P$32 | R9.2 14.45,40.28 v14.45,41.07
  Route2 0.203: v19.84,37.77 19.7,37.61 18.82,37.61 18.56,37.74 17.58,37.74 16.21,39.22 14.5,39.22 14.1,39.6 14.1,40.84 v14.45,41.07
  Bottom 0.203: R11.1 18.95,37.4 19.14,37.36 19.48,37.36 v19.84,37.77
!RST
  Top 0.203: U12.P$7 2.99,34.75 C18.2
A3
  Top 0.203: U12.P$13 4.64,30.57 R14.1 R15.2
A4
  Top 0.203: U12.P$18 7.14,31.2 6.91,30.81 6.91,27.15 3.33,23.75 3.33,21.97 2.92,21.57 2.92,20.14 2.54,19.76 2.54,18.24 2.16,17.86 2.16,16.41 U$14.P$1
A5
  Top 0.203: U12.P$19 7.64,31.2 7.49,30.98 7.49,30.07 U$4.P$1
ANT
  Top 0.406: C10.1 arc90 21.83,40.93 U$15.P$1
BTN
  Top 0.203: U12.P$44 6.64,39.88 R1.2 6.76,40.22 U$10.P$2
CK  (via drill 0.25)
  Top 0.203: U12.P$39 9.14,38.86 v9.2,39.01
  Route2 0.203: v9.2,39.01 9.2,44.37 U$31.P$2
D3  (via drill 0.25)
  Top 0.203: v11.91,32.72 10.8,32.72 U12.P$26
  Route2 0.203: v11.91,32.72 10.9,32.72 9.91,33.5 9.91,37.29 10.74,37.97 11.86,37.97 13.03,39.24 13.03,43.46 U$31.P$1
D4  (via drill 0.25)
  Top 0.203: U12.P$27 11.49,33.25 v11.56,33.19
  Route2 0.203: v11.56,33.19 11.54,33.19 11.43,33.3 10.72,33.3 10.26,33.68 10.26,37.11 10.9,37.64 12.01,37.64 13.39,39.14 13.39,44.6 U$32.P$2
D5  (via drill 0.25)
  Top 0.203: v11.41,33.76 U12.P$28
  Route2 0.203: v11.41,33.76 10.8,33.76 10.62,33.88 10.62,36.93 11.07,37.31 12.17,37.31 13.74,39.04 13.74,43.46 14.99,44.76 15.47,44.76 U$32.P$1
D6  (via drill 0.25)
  Top 0.203: U12.P$45 6.14,38.91 v6.17,39.01
  Route2 0.203: v5.46,40.72 5.46,42.72 U$36.P$1
  Bottom 0.203: v6.17,39.01 6.17,39.65 v5.46,40.72
D8  (via drill 0.25)
  Top 0.203: U12.P$38 9.64,38.85 v9.78,39.01
  Route2 0.203: U$14.P$2 1.17,13.34 2.49,13.34 3.28,14.12 3.28,38.89 4.78,40.13 7.37,40.13 8.69,38.56 9.5,38.56 9.78,38.84 v9.78,39.01
D9
  Top 0.203: U12.P$12 3.84,32.12 3.84,25.66 2.24,24.11 2.24,22.58 U$16.P$2
D10  (via drill 0.25)
  Top 0.203: 15.48,38.96 R2.1 | U12.P$29 11.6,34.25 v11.76,34.24 | 15.49,38.88 v15.49,38.74 v15.49,38.73
  Top 0.254: U1.P$7 15.49,38.88 R2.1
  Route2 0.203: v11.76,34.24 11.25,34.24 10.97,34.47 10.97,36.78 11.2,36.96 12.29,36.96 13.92,38.73 v15.49,38.73
D11
  Top 0.203: U12.P$17 6.64,31.31 6.64,31.19 6.51,30.94 6.51,27.26 2.97,23.88 2.97,22.17 2.52,21.72 2.52,20.3 2.13,19.91 2.13,18.41 U$17.P$2
D12
  Top 0.203: U12.P$16 6.14,27.43 2.62,24 2.62,22.33 2.18,21.89 2.18,20.5 U$17.P$1
D13
  Top 0.203: U12.P$11 3.67,32.75 3.5,32.59 3.5,25.81 U$16.P$1
DM  (via drill 0.25)
  Top 0.203: U12.P$32 11.29,35.75 v11.43,35.79
  Bottom 0.254: RA1.P$1 7.19,35.03 7.7,35.54 D8.P$4 9.48,35.54 9.75,35.79 v11.43,35.79
  Bottom 0.305: RA1.P$1
DP  (via drill 0.25)
  Top 0.203: U12.P$33 11.23,36.25 v11.43,36.37
  Bottom 0.254: RA1.P$2 6.48,35.65 6.48,36.14 6.88,36.54 D8.P$1 9.43,36.54 9.75,36.37 v11.43,36.37
GND  (via drill 0.25)
  Top 0.152: C27.2 15.13,6.43 U11.4
  Top 0.203: U8.P$11 U8.P$10 U8.P$14 9.96,2.49 C8.2 10.52,1.93 10.52,1.08 C22.2 10.35,0.94 11.12,0.94 | U10.11 8.39,8.47 8.08,8.89 C26.2 | U10.9 9.19,8.42 C25.2 | U10.18 7.37,5.32 6.8,5.32 6.45,4.98 | U9.P$5 U9.P$6 | U9.P$8 U9.P$6 | U9.P$4 U9.P$6 | U10.20 8.39,4.3 8.15,4.12 7.52,4.12 7.21,4.42 7.01,4.42 6.45,4.98 | 6.45,4.98 6.43,4.98 6.15,5.26 C24.2 | 10.36,0.84 10.36,0.86 | U1.P$33 16.74,35.53 v16.36,35.15 | 4.97,34.25 5.13,34.09 v5.13,32.46 | 9.64,30.56 C41.1 | 5.03,39.41 C40.1 | 9.88,37.25 v9.12,37.44
  Top 0.254: C3.1 21.56,35.6 U2.P$4 | C4.1 20.46,33.64 U2.P$2 | v9.07,36.04 6.98,37.39 | 5.07,39.15 C40.1 | 5.03,39.41 5.03,38.86 5.16,38.73 5.16,38.41 U12.P$47 | U12.P$35 9.88,37.25 | 9.64,30.56 U12.P$23 9.64,32.83 9.68,32.87 | 9.64,32.45 v8.99,32.46 | U12.P$47 5.14,37.25 5.26,37.13 5.21,37.13 v5.13,37.49 5.18,37.49 5.13,37.54 | U12.P$8 6.64,34.25 v6.76,34.37
  Bottom 0.203: v18.34,34.06 18.41,34.06
  Bottom 0.254: v7.39,36.04 D8.P$5 9.12,36.04
  Bottom 0.406: J1.5 4.88,36.98 5.49,36.98 | C14.2 8.7,28.27 U7.P$2 9.07,29.41 U7.P$5
  other vias: 20.75,23.27 21.87,23.27 17.78,21.01 16.76,23.27 18.82,12.29 19.76,12.29 20.78,12.29 21.87,12.29 14.76,21.01 13.77,23.27 13.72,12.29 12.75,12.29 8.23,19.81 8.23,15.8 17.83,19.79 17.83,18.54 17.83,17.27 17.83,16.05 17.83,14.73 18.01,10.36 16.41,6.15 15.8,7.52 16.81,1.57 3.05,5.26 17.27,36.22 6.68,25.88 22.38,35.41 22.38,34.37 22.38,33.27 22.35,36.5 22.35,37.67 22.35,38.48 21.54,38.51 18.06,40.46 6.3,41.5 16.36,37.26 16.36,36.25 17.32,34.06 17.25,37.26 18.06,37.26 18.34,35.15 16.36,34.06 19.51,40.94 19.53,41.81 19.51,42.67 8.99,33.58 18.8,40.74 22.35,39.12 21.21,39.12 17.48,38.89 17.48,39.8 22.38,32.49 17.78,23.27 18.77,23.34 18.69,39.4 18.59,38.79 16.87,10.36 17.27,35.15 18.08,36.25 7.98,34.8 14.27,38.1 15.16,37.26 5.41,29.39 12.14,40.13 7.65,32.46 7.62,33.66 6.45,37.49 7.39,37.44 5.13,33.66 6.2,32.46 19.79,23.34 18.54,42.67 18.57,41.78 9.04,34.77
  pour Top (isolate 0.203): 0,0 0,39.29 22.99,39.29 23.06,21.49 18.03,21.49 18.03,14.17 22.96,14.17 22.96,0 16,0 16,6.76 12.75,6.76 12.75,3.56 15.95,3.56 15.95,0 10.67,0 10.67,8.03 7.26,8.03 7.26,4.67 10.66,4.67 10.66,0
  pour Route2 (isolate 0.254): 0,0 0,39.27 22.99,39.27 23.04,21.34 18.03,21.34 18.03,14.07 23.04,14.07 22.99,0 10.67,0 10.67,7.98 7.26,8.03 7.26,4.67 10.62,4.67 10.62,0
  pour Bottom (isolate 0.254): 0,0 0,30.25 22.99,30.25 22.99,21.39 18.03,21.39 18.03,14.17 22.99,14.17 22.99,0 10.67,0 10.67,8.03 7.26,8.03 7.26,4.67 10.66,4.67 10.66,0
  pour Bottom (isolate 0.254, no thermals): 0,41.38 0,45.82 19.68,45.82 19.68,30.25 4.85,30.25 4.85,41.38
  pour Bottom (isolate 0.254): 19.7,39.27 22.99,39.27 22.99,25.17 19.7,25.17
  pour Route2 (isolate 0.254): 19.68,39.27 0,39.27 0,45.82 19.68,45.82
  pour Top (isolate 0.254): 0,39.27 0,45.82 19.68,45.82 19.68,39.27
GPIO0  (via drill 0.25)
  Top 0.203: U1.P$15 13.67,34.41 v13.49,34.57
  Route2 0.203: v14.05,32.64 14.2,32.79 18.31,32.79 20.55,31.52 20.55,29.46 21.72,27.71 U$3.P$1
  Bottom 0.203: v13.49,34.57 13.89,34.29 R13.1 14.11,33.04 v14.05,32.64
GPIO2  (via drill 0.25)
  Top 0.203: U1.P$14 13.96,34.91 v13.49,35.15
  Bottom 0.203: v13.49,35.15 13.52,35.1 R3.1
GPIO15  (via drill 0.25)
  Top 0.203: U1.P$13 13.97,35.41 v13.49,35.76
  Bottom 0.203: R6.2 13.95,36.14 v13.49,35.76
GPIO16
  Top 0.203: U1.P$8 14.99,38.64 R9.1
N$1
  Top 0.254: U1.P$28 20.16,35.41 U2.P$1 20.46,35.62 C3.2
N$2
  Top 0.152: 21.5,34.2 21.03,34.67 19.91,34.67
  Top 0.254: C4.2 21.56,33.64 U2.P$3 21.5,34.2 | 19.91,34.67 19.51,34.9 U1.P$27
N$3
  Top 0.254: U1.P$2 17.99,39.35 arc-90 18.77,40.01 C10.2
N$4
  Bottom 0.254: D4.P$2 SJ2.1
N$5
  Bottom 0.254: R12.2 D4.P$1
N$6
  Top 0.254: U3.P$7 15.77,12.1 L2.1
N$8
  Top 0.203: R18.2 U$2.P$2
N$9
  Top 0.203: C34.2 0.94,37.25 X2.P$2 2.73,36.75 U12.P$3
N$10
  Top 0.254: U3.P$6 14.77,12.27 L7.1
N$11
  Top 0.203: U$4.P$2 R16.2
N$12
  Top 0.203: C35.2 0.92,35.75 X2.P$1 2.74,36.25 U12.P$4
N$13
  Top 0.203: 20.4,37.55 19.76,36.93 19.16,36.93
  Top 0.254: R4.1 20.4,37.55 | 19.16,36.93 U1.P$31
N$17
  Top 0.203: U12.P$9 3.14,33.75 C36.2 C37.2 L9.2
N$19  (via drill 0.25)
  Top 0.203: U8.P$16 9.08,3.41 v8.59,3.86 | v6.78,8.36 7.93,8.36 7.99,8.32 U10.12
  Route2 0.203: v6.78,8.36 6.38,8.36 6.17,8.18 6.17,4.52 6.45,4.32 7.19,4.32 7.62,3.86 v8.59,3.86
N$23
  Top 0.254: U3.P$3 L8.1
N$26
  Top 0.203: U8.P$15 9.86,2.89 C8.1
N$31
  Bottom 0.254: J1.3 5.49,35.68 RA1.P$4
N$33
  Bottom 0.254: J1.2 RA1.P$3
N$40
  Top 0.203: U10.10 8.79,9.05 C26.1
N$43
  Top 0.254: U3.P$25 10.77,23.4 10.84,23.42 L4.2
N$44
  Top 0.254: U3.P$26 9.77,23.41 9.78,23.48 L5.2
N$45
  Top 0.254: U3.P$17 U3.P$16
N$46
  Top 0.254: U3.P$23 12.79,23.57 R10.2
N$47
  Top 0.254: U3.P$29 8.25,17.78 L6.1
PPS  (via drill 0.25)
  Top 0.203: v2.79,17.78 5.87,17.78 | 5.87,17.78 L6.2 | 3.93,37.26 U12.P$2 3.49,37.25 3.3,37.44 3.3,37.77 3,38.08 v2.62,38.08 | U$2.P$1 5.87,17.78
  Route2 0.203: v2.62,38.08 2.77,38.08 2.92,37.8 2.92,18.01 v2.79,17.78
PWRIN
  Bottom 0.305: D2.P$1 8.67,30.02 U7.P$3 8.7,30.31 8.91,30.52 9.45,30.52 | C11.1 9.45,30.52 | U7.P$4 9.44,30.51 9.45,30.52
  Bottom 0.406: D2.P$1 D1.P$1
RX2  (via drill 0.25)
  Top 0.203: U1.P$26 19.54,34.41 19.68,34.24 v19.68,33.3 | U12.P$31 11.43,35.26 v11.73,35.26
  Route2 0.203: U$1.P$1 21.77,31.47 21.77,31.65 19.68,32.84 v19.68,33.3 19.46,33.45 13.97,33.45 12.78,34.34 12.78,34.82 12.34,35.26 v11.73,35.26
RXDD  (via drill 0.25)
  Top 0.203: L5.1 9.41,24.58 v9.07,24.74 8.64,25.07 8.64,31.19 8.64,31.29 U12.P$21
  Route2 0.203: v5.84,12.5 5.05,13.46 5.05,23.72 6.17,24.84 8.97,24.84 v9.07,24.74 | U$12.P$2 2.08,4.34 4.06,4.34 4.39,4.65 4.39,9.25 v4.27,9.35
  Bottom 0.203: v5.84,12.5 5.84,12.47 5.31,11.94 5.31,10.11 4.55,9.35 v4.27,9.35 4.24,9.35
SCL  (via drill 0.25)
  Top 0.203: U8.P$5 8.28,1.93 8.05,1.7 7.01,1.7 v6.76,1.91 | v13.77,10.21 14.56,10.21 R7.1 | U12.P$42 7.62,38.4 7.62,38.94 v7.7,39.01
  Top 0.254: L7.2 R7.1
  Route2 0.203: 5.46,10.01 4.46,11.44 3.61,11.44 | 5.46,10.01 5.46,3.17 6.68,1.96 v6.76,1.91 | 5.46,10.01 13.59,10.01 v13.77,10.21 | v7.7,39.01 7.14,39.8 4.9,39.8 3.63,38.73 3.63,12.28 3.49,12.06 3.49,11.56 3.61,11.44 | 3.61,11.44 2.65,11.44 2.52,11.3 2.52,10.08 2.16,9.73 2.16,8.28 U$12.P$1
SCL2  (via drill 0.25)
  Top 0.203: U8.P$8 8.28,3.5 8.03,3.76 7.06,3.76 v7.01,3.81 6.66,4.16 RA2.P$1 | U9.P$3 14.48,3.18 | 14.48,3.18 U11.3 | 14.48,3.18 14.55,3.18 v14.58,3.25 | v9.8,3.96 9.6,4.22 9.6,4.71 U10.23
  Route2 0.203: v14.58,3.25 9.8,3.25 | 9.8,3.25 v9.8,3.96 | v7.01,3.81 7.01,3.71 7.42,3.25 9.8,3.25
SDA  (via drill 0.25)
  Top 0.203: U8.P$1 7.43,2.09 v7.19,2.34 | v7.11,39.01 7.14,38.86 U12.P$43
  Top 0.254: R8.1 L8.2 11.44,10.98 v10.92,10.46
  Route2 0.203: 10.77,10.49 v10.92,10.46 v7.16,10.46 5.61,10.46 4.55,11.91 v3.99,11.91 3.99,38.58 5.03,39.47 6.86,39.47 v7.11,39.01 | v7.19,2.34 7.04,2.34 5.82,3.38 5.82,8.43 6.4,8.91 v7.01,8.91 | v2.95,11.91 2.41,11.91 2.16,11.66 2.16,10.31 U$13.P$2
  Bottom 0.203: v7.01,8.91 6.96,8.97 7.16,9.17 v7.16,10.46 | v2.95,11.91 v3.99,11.91
SDA2  (via drill 0.25)
  Top 0.203: U8.P$4 6.86,3.29 | 13.24,3.96 U11.2 14.05,3.51 U9.P$2 14.04,2.54 v13.46,2.54 | 6.86,3.29 6.86,3.26 v6.86,3.15 | RA2.P$2 6.55,3.56 6.86,3.29 | U10.24 9.99,4.49 10.31,4.17 10.31,4.06 10.52,3.86 10.82,3.86 10.92,3.76 10.92,2.9 v11.02,2.79
  Route2 0.203: v13.46,2.54 13.21,2.9 11.02,2.9 | 11.02,2.9 7.11,2.9 v6.86,3.15 | v11.02,2.79 11.02,2.9
SI  (via drill 0.25)
  Top 0.203: U12.P$41 8.14,38.75 8.23,38.86 v8.23,39.83
  Route2 0.203: v8.23,39.83 8.23,43.28 7.8,43.69 6.38,43.69 U$30.P$2
SINT  (via drill 0.25)
  Top 0.203: U8.P$9 v8.68,1.6 v8.69,1.6 | v5.59,39.01 5.64,38.89 U12.P$46
  Route2 0.203: v8.69,1.6 8.64,1.6 8.41,1.45 6.53,1.45 5.11,2.95 5.11,9.88 4.65,10.54 v4.39,10.54 | v4.52,12.47 4.34,12.7 4.34,38.43 5,39.01 v5.59,39.01
  Bottom 0.203: v4.39,10.54 4.52,10.62 v4.52,12.47
SO  (via drill 0.25)
  Top 0.203: U12.P$40 8.64,39.17 v8.74,39.4
  Route2 0.203: v8.74,39.4 8.74,43.38 U$30.P$1
TX2  (via drill 0.25)
  Top 0.203: U1.P$25 19.05,33.86 19.05,33.01 v19.07,32.99 | U12.P$30 11.32,34.75 v11.43,34.75
  Route2 0.152: 21.84,29.41 U$1.P$2
  Route2 0.203: 21.84,29.41 20.9,30.63 20.9,31.73 19.07,32.78 v19.07,32.99 18.97,33.12 13.82,33.12 12.42,34.16 12.42,34.57 12.22,34.75 v11.43,34.75
TXDD  (via drill 0.25)
  Top 0.203: L4.1 10.87,24.94 v10.87,25.2 9.4,25.2 9.07,25.48 9.07,31.19 9.14,31.32 U12.P$22
  Route2 0.203: v10.87,25.2 6.05,25.2 4.7,23.85 4.7,13.31 v5.16,12.47 | v4.47,9.96 4.75,9.6 4.75,4.5 4.18,4 2.07,4 U$11.P$1
  Bottom 0.203: v4.47,9.96 4.9,10.31 4.9,12.01 v5.16,12.47
USB_SHIELD1
  pour Bottom (isolate 0.254, rank 3, no thermals): 0,41.17 4.7,41.17 4.7,30.25 0,30.25
VBAT  (via drill 0.25)
  Top 0.203: R14.2 5.48,30.56 v5.41,30.54
  Bottom 0.152: v5.41,30.54 5.35,30.54
  Bottom 0.203: 5.35,30.54 5.53,30.54 5.99,30.07 5.99,28.8 5.94,28.75
  Bottom 0.254: 2.54,28.75 2.96,28.75 | 4.9,28.7 4.85,28.75
  Bottom 0.406: D1.P$2 6.88,28.85 6.71,28.75 5.94,28.75 4.85,28.75 2.54,28.75 1.58,28.75 JP9.1
VBATRTC
  Top 0.203: U12.P$1 3.85,37.75 3.2,38.41 3.2,42.85 2.97,43.08 2.92,43.08 U$36.P$2
VBBAT  (via drill 0.25)
  Top 0.254: U3.P$8 16.77,12.18 C29.1 v16.87,11.81
  Bottom 0.254: v16.87,11.81 18.31,10.9 19.24,10.9 R12.1 19.26,9.16 U4.P$1
VBUS  (via drill 0.25)
  Top 0.203: U12.P$20 8.14,30.98 v7.95,30.79
  Bottom 0.203: v7.95,30.79 7.12,30.79 6.94,30.96
  Bottom 0.406: D2.P$2 6.94,30.96 6.94,32.92 5.87,34.38 J1.1
VDD  (via drill 0.25, 0.33)
  Top 0.203: U8.P$13 9.25,1.75 C22.1 | C22.1 9.2,0.97 v9.8,1.63 | U10.22 v9.2,3.96 | U11.1 13.43,6.92 C27.1 14.03,7.78 v14.58,8.51 | v16.76,2.69 16.81,2.68 C23.1 16.05,2.53 U9.P$1 | v4.65,3.56 RA2.P$4 RA2.P$3 | R8.2 10.96,9.13 C25.1 10.05,8.53 9.7,8.53 9.59,8.42 U10.8 | v6.2,9.42 6.2,7.26 C24.1 6.17,7.35 U10.13 | U10.1 11.95,5.35 v11.99,5.38 | C20.1 C22.1 | C28.1 13.23,36.74 | L9.1 1.76,30.65 v2.03,30.38 | C39.2 11.04,39.43 | U$10.P$3 11.05,40.77 v11.05,40.13
  Top 0.254: U3.P$9 17.79,12.4 C7.1 18.18,11.88 v18.69,11.53 | R7.2 14.59,8.75 v14.58,8.51 | R8.2 v11.79,8.51 | U3.P$1 9.77,12.09 C30.1 9.11,12.08 v8.94,12.09 | 11.04,39.43 v11.05,40.13 | v3.73,40.34 3.86,39.76 C40.2 4.64,38.6 U12.P$48 | C39.2 11.06,37.83 11.02,37.74 U12.P$36
  Top 0.305: U1.P$3 U1.P$4 16.99,38.46 16.66,38.79 C9.1 16.64,39.3 16.52,39.48 R2.2 | U1.P$30 19.49,36.41 v19.79,36.17 19.5,35.91 U1.P$29 | U1.P$1 19.06,38.06 v19,38.08 19.36,38.38 C2.1 | 15.43,40.45 v15.44,41.06 | C1.1 C5.1 | C5.1 v14.28,31.47 14.99,32.16 | U1.P$11 13.56,36.41 C28.1 | 13.23,36.74 v12.9,36.07 | U12.P$24 10.14,31.25 C41.2 C38.2 10.69,28.41 v10.14,27.86 | U1.P$17 14.99,32.35 C5.1
  Top 0.406: R2.2 15.43,40.45
  Route15 0.203: v9.8,1.63 9.7,1.47 | v9.2,3.96 9.25,3.96 | v16.76,2.69 16.82,2.64 | v4.65,3.56 4.78,3.56 | v6.2,9.42 6.2,9.14 | v11.99,5.38 11.94,5.38 11.89,5.33 | v12.9,36.07 13.34,36.73 | v14.28,31.47 14.58,31.37 | v2.03,30.38 1.8,30.63
  Route15 0.254: 18.47,11.61 v18.69,11.53 | v14.58,8.51 14.58,8.64 | v11.79,8.51 11.76,8.84 | v8.94,12.09 8.97,12.01 8.91,12.06 8.91,12.09 8.87,12.14 | v21.46,7.32 21.46,7.14 21.49,7.11 | v11.05,40.13 11.07,39.52 | v3.73,40.34 3.86,39.93
  Route15 0.305: v15.44,41.06 15.44,40.51
  Route15 0.406: v10.14,27.86 9.63,27.86
  Bottom 0.203: v19.79,36.17 19.32,36.17 R11.2 | R3.2 R13.2 15.23,32.38 v14.28,31.47
  Bottom 0.254: SJ2.2 v21.46,7.32
  Bottom 0.305: U7.P$1 9.44,28.4 C14.1 9.53,27.86
  Bottom 0.406: 9.53,27.86 v10.14,27.86
  pour Route15 (isolate 0.254, no thermals): 0.64,0.64 0.64,39.27 22.43,39.27 22.35,22.02 17.5,22.02 17.5,13.49 22.35,13.49 22.35,0.64 10.62,0.64 10.62,8.03 7.26,8.03 7.26,4.67 10.57,4.67 10.57,0.64
  pour Route15 (isolate 0.254): 0.64,39.27 0.64,45.19 19.68,45.19 19.68,39.27
WAKEUP  (via drill 0.25)
  Top 0.203: L2.2 15.72,10.31 v15.75,10.29 | v11.41,32.26 11.28,32.25 11.02,32.25 U12.P$25
  Route2 0.203: v15.75,10.29 15.37,10.29 14.96,10.69 11.43,10.69 11.07,10.92 6.86,10.92 6.38,11.4 6.38,12.65 5.41,13.61 5.41,23.6 6.3,24.49 8.59,24.49 8.79,24.28 9.4,24.28 9.8,24.71 11.43,24.71 11.61,25.09 11.61,31.95 v11.41,32.26

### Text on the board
tPlace: VB | D6 | D24 | D22 | D23 | D3 | D4 | D5 | GND | STM32L4 | BTN | ESP8285 | RST | TX2 | RX2 | + | 00 | - | Asset Tracker | D13 | D9 | D12 | D11 | A4 | CAM M8Q | D8 | 3V3 | SDA | EM7180 | MPU9250 | SCL | TX1 | RX1 | Ay,Mx | GND
bPlace: v.02b | Pesky / Products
